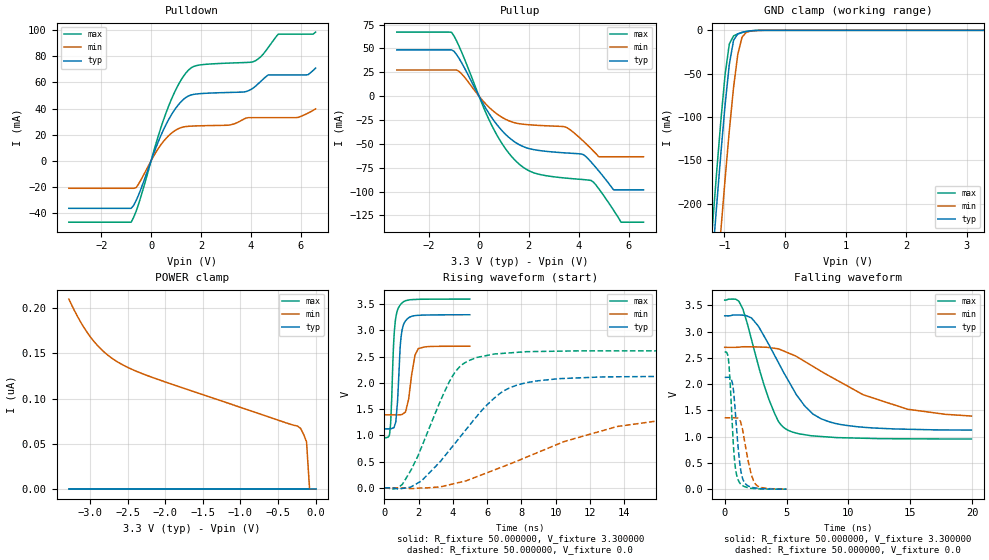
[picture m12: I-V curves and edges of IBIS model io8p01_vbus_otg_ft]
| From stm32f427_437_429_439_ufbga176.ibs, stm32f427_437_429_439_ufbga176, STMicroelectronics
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|   Model io8p01_vbus_otg_ft
[Model]  io8p01_vbus_otg_ft
Model_type I/O
Polarity   Non-Inverting
Enable   Active-Low
Vinl =   0.990000V
Vinh =   2.310000V
Vmeas =  1.650000V
Cref =   50.000000pF
Rref =   100.000000M
Vref =   0.0V
C_comp   3.304800pF   3.199300pF   3.429300pF
[Temperature Range]   25.000000   0.125000k   -40.000000
[Pullup Reference]   3.300000V   2.700000V   3.600000V
[Pulldown Reference]   0.0V   0.0V   0.0V
[POWER Clamp Reference]   3.300000V   2.700000V   3.600000V
[GND Clamp Reference]   0.0V   0.0V   0.0V
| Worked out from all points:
|   slope of the pulldown table from 0 to 0.495 V, typ, clamps not added: 20.9 ohm
|   slope of the pullup table from 0 to 0.495 V, typ, clamps not added: 22.6 ohm
|   GND clamp passes 1 mA (typ) near -0.61 V on its own axis
|   rising waveform, R_fixture 50.000000, V_fixture 3.300000: 20-80 % time 225ps typ, 351ps min, 207ps max; typ from 1.12 V to 3.3 V
|   rising waveform, R_fixture 50.000000, V_fixture 0.0: 20-80 % time 3.35ns typ, 6.83ns min, 2.07ns max; typ from 0 V to 2.13 V
|   falling waveform, R_fixture 50.000000, V_fixture 3.300000: 20-80 % time 3.27ns typ, 6.64ns min, 2.04ns max; typ from 3.3 V to 1.12 V
|   falling waveform, R_fixture 50.000000, V_fixture 0.0: 20-80 % time 481ps typ, 679ps min, 387ps max; typ from 2.13 V to 0 V
[Pulldown]
|Voltage   I(typ)   I(min)   I(max)
-3.3V     -36.41mA   -21.08mA   -47.04mA
-800mV    -36.41mA   -21.08mA   -47.04mA
-600mV    -30.48mA   -20.53mA   -38.65mA
700mV     31.4mA     19.11mA    41.71mA
1.2V      45.15mA    25.37mA    61.75mA
1.6V      50.35mA    26.5mA     71.06mA
3.1V      52.28mA    27.26mA    74.76mA
4.1V      55.7mA     33mA       75.81mA
4.7V      65.72mA    33mA       86.7mA
5.1V      65.72mA    33mA       96.91mA
6.3V      65.88mA    36.51mA    96.91mA
6.6V      70.94mA    39.72mA    98.51mA
[Pullup]
|Voltage   I(typ)   I(min)   I(max)
-3.3V     48.54mA    27.44mA    67.18mA
-1.1V     48.54mA    27.44mA    66.9mA
-700mV    35.13mA    23.47mA    46.35mA
500mV     -22.07mA   -14mA      -30.03mA
1.5V      -49.1mA    -28.3mA    -68.56mA
2.2V      -56.05mA   -30.32mA   -80.35mA
3.5V      -59.53mA   -32.66mA   -85.92mA
4.5V      -69.06mA   -55.13mA   -88.4mA
4.8V      -78.23mA   -63.5mA    -96.84mA
5.4V      -98.2mA    -63.5mA    -119.6mA
5.7V      -98.2mA    -63.5mA    -132.1mA
6.6V      -98.2mA    -63.5mA    -132.1mA
[GND_clamp]
|Voltage   I(typ)   I(min)   I(max)
-3.3V     -2.321A    -2.399A    -2.294A
-1.2V     -265.6mA   -356.2mA   -227.3mA
-1.13V    -202.8mA   -293mA     -164.3mA
-1.06V    -142.3mA   -231.2mA   -104.3mA
-990mV    -86.15mA   -171.7mA   -51mA
-920mV    -39.05mA   -115.6mA   -15.71mA
-850mV    -11.4mA    -65.74mA   -6.366mA
-780mV    -4.046mA   -27.6mA    -4.153mA
-710mV    -2.285mA   -7.882mA   -2.591mA
-640mV    -1.291mA   -2.274mA   -1.367mA
-570mV    -618uA     -909.9uA   -567.3uA
3.28V     0A         0A         0A
[POWER_clamp]
|Voltage   I(typ)   I(min)   I(max)
-3.28V    0A         210.1nA    0A
-3.12V    0A         184.2nA    0A
-2.96V    0A         164.6nA    0A
-2.8V     0A         150.7nA    0A
-2.6V     0A         139nA      0A
-2.16V    0A         123.2nA    0A
-240mV    0A         69.7nA     0A
-200mV    0A         67.32nA    0A
-160mV    0A         60.72nA    0A
-120mV    0A         52.23nA    0A
-80mV     0A         0A         0A
0V        0A         0A         0A
[Ramp]
| variable   typ   min   max
dV/dt_r  1.27764/3.34799n   0.79902/6.85385n   1.56780/2.07214n
dV/dt_f  1.30254/3.27846n   0.73944/6.61301n   1.58786/2.04132n
R_load = 50.000000
[Rising Waveform]
R_fixture= 50.000000
V_fixture= 3.300000
V_fixture_min= 2.700000
V_fixture_max= 3.600000
|time   V(typ)   V(min)   V(max)
0s        1.124V     1.392V     954.4mV
300.3ps   1.126V     1.392V     1.026V
370.4ps   1.127V     1.392V     1.285V
580.6ps   1.172V     1.392V     2.989V
670.7ps   1.28V      1.391V     3.26V
850.9ps   2.213V     1.392V     3.451V
930.9ps   2.736V     1.394V     3.49V
1.101ns   3.1V       1.415V     3.545V
1.982ns   3.289V     2.655V     3.594V
4.985ns   3.3V       2.7V       3.599V
[Rising Waveform]
R_fixture= 50.000000
V_fixture= 0.0
V_fixture_min= 0.0
V_fixture_max= 0.0
|time   V(typ)   V(min)   V(max)
0s        358uV      202.4uV    672.5uV
1.081ns   -9.476mV   -1.93mV    83.55mV
2.162ns   131.5mV    -2.594mV   771.8mV
3.804ns   719.5mV    59.22mV    2.031V
4.284ns   914.1mV    95.97mV    2.269V
4.885ns   1.158V     147.5mV    2.42V
6.807ns   1.815V     389.5mV    2.561V
8.288ns   2.003V     583.7mV    2.596V
13.61ns   2.117V     1.17V      2.611V
19.94ns   2.129V     1.359V     2.612V
[Falling Waveform]
R_fixture= 50.000000
V_fixture= 3.300000
V_fixture_min= 2.700000
V_fixture_max= 3.600000
|time   V(typ)   V(min)   V(max)
0s        3.3V       2.7V       3.599V
880.9ps   3.315V     2.7V       3.615V
1.441ns   3.312V     2.71V      3.442V
2.162ns   3.26V      2.71V      2.851V
3.604ns   2.737V     2.695V     1.691V
5.045ns   2.106V     2.603V     1.131V
6.486ns   1.578V     2.429V     1.036V
8.488ns   1.279V     2.15V      991.2mV
14.73ns   1.141V     1.524V     958.7mV
19.94ns   1.124V     1.392V     954.4mV
[Falling Waveform]
R_fixture= 50.000000
V_fixture= 0.0
V_fixture_min= 0.0
V_fixture_max= 0.0
|time   V(typ)   V(min)   V(max)
0s        2.129V     1.359V     2.612V
300.3ps   2.13V      1.359V     2.477V
620.6ps   2.02V      1.358V     1.201V
810.8ps   1.616V     1.36V      518.2mV
1.111ns   736.3mV    1.344V     163.1mV
1.301ns   355.5mV    1.266V     94.58mV
1.522ns   159.7mV    1.031V     58.14mV
2.142ns   39.61mV    284.5mV    16.4mV
2.452ns   24.17mV    108mV      10.87mV
4.985ns   358uV      202.4uV    672.5uV
